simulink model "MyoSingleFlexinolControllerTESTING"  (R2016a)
settings: Solver=FixedStepAuto  StartTime=0.0  StopTime=10.0  RelTol=1e-3
libraries: arduinolib x4

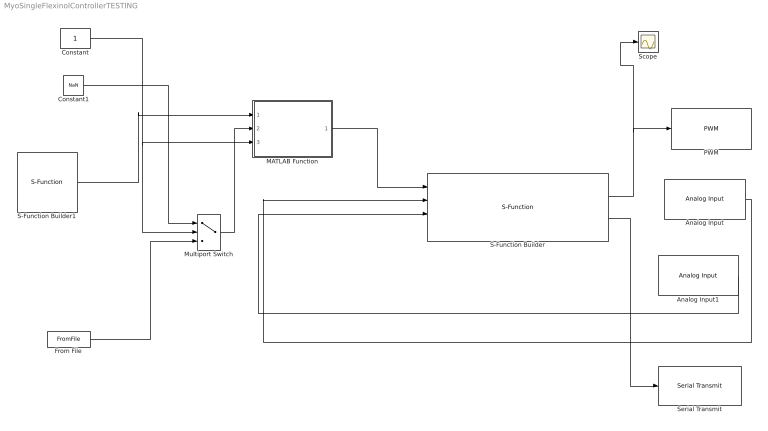
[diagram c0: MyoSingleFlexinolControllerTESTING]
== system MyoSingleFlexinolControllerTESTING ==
  Analog Input : arduinolib/Analog Input  pinNumber=1  sampleTime=1  blockPlatform=arduino
  Analog Input1 : arduinolib/Analog Input  pinNumber=0  sampleTime=1  blockPlatform=arduino
  Constant : Constant  OutMin=0  OutMax=1
  Constant1 : Constant  Value=NaN
  From File : FromFile  FileName=MatrixesForNN.mat  SampleTime=0
  MATLAB Function : MATLAB Function  TreatAsAtomicUnit=on
  Multiport Switch : MultiPortSwitch  DataPortOrder=Zero-based contiguous  Inputs=2  OutMin=0  OutMax=1  OutDataTypeStr=single
  PWM : arduinolib/PWM  pinNumber=5  blockPlatform=arduino
  S-Function Builder : S-Function  InitFcn=try, set_param(gcb,'FunctionName','actuateFlexinol'), end  FunctionName=actuateFlexinol  SFunctionModules=actuateFlexinol_wrapper  SFunctionDeploymentMode=off  EnableBusSupport=off
  S-Function Builder1 : S-Function  InitFcn=try, set_param(gcb,'FunctionName','readEMG'), end  FunctionName=readEMG  SFunctionModules=readEMG_wrapper  SFunctionDeploymentMode=off  EnableBusSupport=off
  Scope : Scope
  Serial Transmit : arduinolib/Serial Transmit  portNumber=0  blockPlatform=arduino
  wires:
  S-Function Builder/1 -> Scope/1, PWM/1
  Analog Input/1 -> S-Function Builder/2
  Analog Input1/1 -> S-Function Builder/3
  S-Function Builder/2 -> Serial Transmit/1
  MATLAB Function/1(y) -> S-Function Builder/1
  Constant/1 -> MATLAB Function/3(clsd), Multiport Switch/2
  S-Function Builder1/1 -> MATLAB Function/1(x_in)
  From File/1 -> Multiport Switch/3
  Multiport Switch/1 -> MATLAB Function/2(t)
  Constant1/1 -> Multiport Switch/1

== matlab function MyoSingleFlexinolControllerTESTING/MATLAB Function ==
function y = NNEMG(x_in, t,clsd) 
persistent indx;
persistent trainFcn;  % Bayesian Regularization backpropagation.%
persistent inputDelays;
persistent feedbackDelays;
persistent hiddenLayerSize;
persistent net;
persistent xfo;
persistent last_t;
persistent afo;%for saving net state after running/training steps
persistent delaySize;
delaySize = 4;
%mlock
persistent x;

%x = [x;u]
if(not(isequal(x_in,[]) && isequal(x_in,x(size(x,1),:))))
    %we suppose that emg signal never can be equal, anywaay euql states do not needs computation
   
    disp('espando il vettore samples set');
    if(isempty(x))
        x = x_in;
    else
        x = [x,x_in];
    end
end

if(isequal(indx,[]))
    disp('inizializzo narnx');
    indx = 0
    %persistent trainFcn;  % Bayesian Regularization backpropagation.
    trainFcn = 'trainbr';
    % Create a Nonlinear Autoregressive Network with External Input
    
    %persistent inputDelays;
    inputDelays = 1:delaySize;
    %persistent feedbackDelays;
    feedbackDelays = 1:delaySize;
    %persistent hiddenLayerSize;
    hiddenLayerSize = 10;
    %persistent net;
    net = narxnet(inputDelays,feedbackDelays,hiddenLayerSize,'open',trainFcn);
    
    % Choose Input and Feedback Pre/Post-Processing Functions
    net.inputs{1}.processFcns = {'removeconstantrows','mapminmax'};
    net.inputs{2}.processFcns = {'removeconstantrows','mapminmax'};
    
    
    
    % Choose a Performance Function
    % For a list of all performance functions type: help nnperformance
    net.performFcn = 'mse';  % Mean Squared Error
    net.name = [net.name ' - open'];
    disp('size:');
     net.inputs{:}.size
     net.inputs{1}.size
    % Choose Plot Functions
    % For a list of all plot functions type: help nnplot
    %net.plotFcns = {'plotperform','plottrainstate', 'ploterrhist', ...
    %  'plotregression', 'plotresponse', 'ploterrcorr', 'plotinerrcorr'};
    
    
end

%for each function call put the array in a input signal matrix,
%then if the matrix is full test the condition 'clsd' and run preparets and
%corrispective nnet(this must preserve his state along varius function
%calls
if(size(x,2) == delaySize+1 )%+1
        indx = indx + 1
        X = x; %X = tonndata(x,true,true)
        x = []; %empty the buffer matrix for next function call
    if(not(clsd))
        
       
        
        
        T = tonndata(t((delaySize)*indx-(delaySize-1):((delaySize)*indx)+1),true,true)%t((delaySize)*indx-((delaySize):(delaySize)*indx:(delaySize)  next delaySize row of the trining result dataset t
        last_t = T;
        %X = num2cell(X)
        % view(net)
        
        
        [x1,xf,af,ts] = preparets(net,X,{},T);
        %[y,xfo,afo] = net(x1,xio,aio);
        [net,y,E,xfo,afo] = adapt(net,x1,ts,xf,af);
        
        disp('dopo adapt ho afo: ');
        last_t = [last_t(2:size(last_t,2)),y];
        afo
        assignin('base','Y',y)
         
    else
        
        
        % Next the the network and its final states will be converted to
        % closed-loop form to make  predictions with only the  inputs
        % provided.
        if(isequal(net.name,['NARX Neural Network - open']))
            [net] = closeloop(net);%[net,xic,aic] = closeloop(net,xfo,afo);
            net.name = ['NARX Neural Network - closed'];
            [x2,xic,aic,ts] = preparets(net,X,{},last_t);
           
            [y,xfo,afo] = net(x2,xic,aic); %adapt(net);
            last_t = [last_t(2:size(last_t,2)),y]; 
        
        %multiStepPerformance = perform(net,T(1,predictOutputTimesteps),y2)
        else
            disp('valore ottenuto da loop chiuso oltre la prima simulazione:');
            x2 = preparets(net,X);
            [y,xfo,afo] = net(x2,xfo,afo);
            y
            last_t = [last_t(2:size(last_t,2)),y]; 
        end
    end
end
